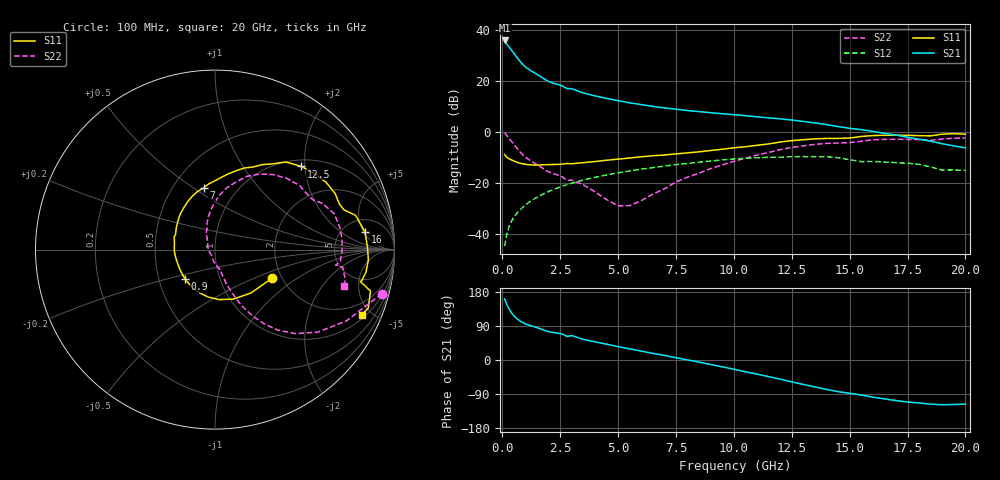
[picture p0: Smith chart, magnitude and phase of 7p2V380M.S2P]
! Infineon Technologies  Discrete & RF Semiconductors
! bfp620
! VCE =  2.3 V,  IC =  80 mA
! Common Emitter S-Parameters:  Sep 2002
# GHz  S  MA  R  50
!  f  S11  S21  S12  S22
! GHz  MAG  ANG  MAG  ANG  MAG  ANG  MAG  ANG
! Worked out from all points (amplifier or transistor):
!   59 points, 100 MHz to 20 GHz, reference 50 ohm
!   highest |S21| = 35.8 dB at 100 MHz (marker M1)
!   |S21| within 3 dB of that: start of sweep to 332.2 MHz
!   unconditionally stable (mu >= 1): 1.972 GHz to 9.858 GHz; 17.18 GHz to end of sweep
!   at 1 GHz: K = 0.89, MSG = 27.1 dB, |S12| = -28.8 dB
!   at 5.5 GHz: K = 1.04, MAG = 12.1 dB, |S12| = -15.4 dB
!   at 20 GHz: K = 1.24, MAG = 1.5 dB, |S12| = -15.2 dB
!   S11 on the Smith chart (normalised r, x): 100 MHz: 1.78, -0.65; 900 MHz: 0.68, -0.24; 7 GHz: 0.70, +0.55; 12.5 GHz: 1.14, +1.92; 16 GHz: 7.89, +5.36; 20 GHz: 1.20, -4.37
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0.1  0.3555 -26.7  61.51 161.4  0.0057 81.0  0.9613 -14.8
0.2  0.3138 -50.6  52.24 145.8  0.0101 75.0  0.833 -28.5
0.3  0.2939 -69.8  45.49 133.6  0.0141 72.5  0.7339 -38.8
0.4  0.2795 -85.4  39.7 124.2  0.0177 71.1  0.6462 -46.4
0.5  0.2666 -98.5  34.51 116.8  0.021 70.1  0.5665 -52.2
0.6  0.2552 -109.8  29.94 110.7  0.0242 69.4  0.4959 -56.5
0.7  0.2459 -119.6  26.08 105.7  0.0273 68.9  0.4359 -59.8
0.8  0.2387 -128.1  22.96 101.6  0.0304 68.5  0.3869 -62.4
0.9  0.2332 -135.3  20.52 98.2  0.0334 68.1  0.3481 -64.3
1.2  0.2241 -151.2  16.05 91.1  0.0426 66.7  0.2744 -67.7
2  0.2266 -179.2  9.679 74.6  0.0672 61.2  0.1637 -73.1
2.8  0.2382 163.0  6.992 62.1  0.0917 54.6  0.1112 -77.1
3  0.2355 159.2  6.972 64.6  0.0979 52.8  0.1123 -76.4
3.5  0.2475 150.6  5.746 54.3  0.1128 48.1  0.0913 -83.6
5  0.2897 127.3  4.048 35.3  0.1563 33.8  0.0353 -127.5
7  0.3494 100.5  2.929 12.1  0.2119 14.6  0.0757 124.7
10.5  0.5071 65.2  2.054 -31.1  0.3011 -24.8  0.303 85.3
12.5  0.6683 43.9  1.694 -57.7  0.3237 -48.4  0.491 59.1
13.5  0.7233 31.3  1.484 -71.1  0.3243 -61.2  0.5638 44.7
16  0.8409 6.8  1.017 -98.1  0.2602 -85.2  0.6942 16.7
17  0.8562 -3.8  0.858 -107.0  0.2477 -93.3  0.7101 4.2
20  0.8943 -24.1  0.482 -116.4  0.1744 -102.7  0.7484 -15.8
